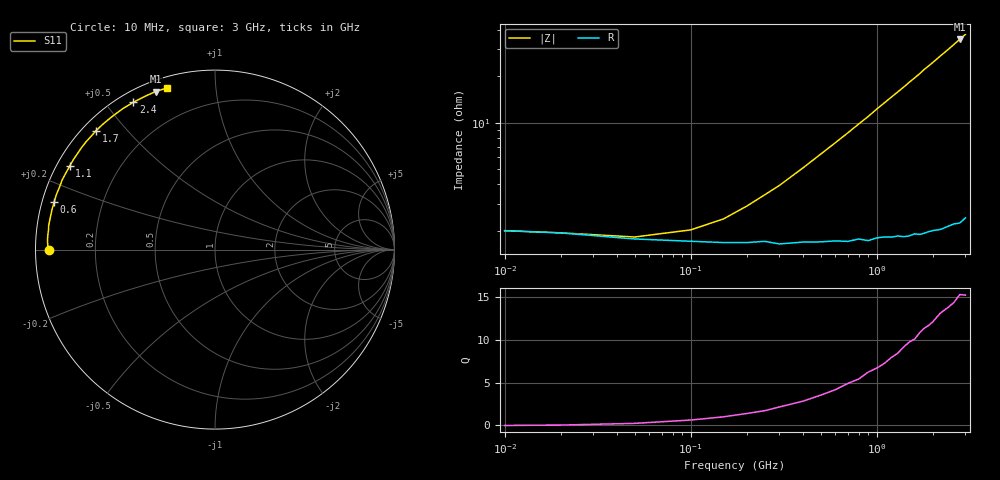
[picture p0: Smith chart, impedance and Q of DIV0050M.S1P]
! SIEMENS Small Signal Semiconductors
! BAV99
! Silicon Switching Diode in SOT23
! IF = 50 mA
! S-Parameters:  May  1995
# GHz  S  MA  R  50
!  f  S11
! GHz  MAG  ANG
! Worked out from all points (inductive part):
!   30 points, 10 MHz to 3 GHz, reference 50 ohm
!   read as one part to ground: L = 1.92 nH near 500 MHz
!   highest Q = 15.3 at 2.8 GHz (marker M1), where L = 1.97 nH
!   S11 on the Smith chart (normalised r, x): 10 MHz: 0.04, +0.00; 600 MHz: 0.03, +0.14; 1.1 GHz: 0.04, +0.27; 1.7 GHz: 0.04, +0.41; 2.4 GHz: 0.04, +0.59; 3 GHz: 0.05, +0.74
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0.01  0.9226 180.0
0.02  0.9251 179.8
0.05  0.9313 179.0
0.15  0.9348 176.1
0.2  0.9349 174.6
0.25  0.9338 173.2
0.3  0.9363 171.8
0.4  0.9349 169.0
0.5  0.935 166.2
0.6  0.9345 163.5
0.7  0.9354 160.8
0.8  0.9337 158.1
0.9  0.9358 155.5
1  0.934 152.7
1.1  0.9338 150.1
1.2  0.9348 147.5
1.4  0.9361 142.5
1.5  0.9363 139.9
1.6  0.9354 137.5
1.7  0.937 135.1
1.8  0.9372 132.4
1.9  0.9368 130.2
2  0.937 127.9
2.2  0.9385 123.3
2.4  0.9384 119.0
2.6  0.9388 114.7
2.8  0.9408 110.6
3  0.9392 106.7
